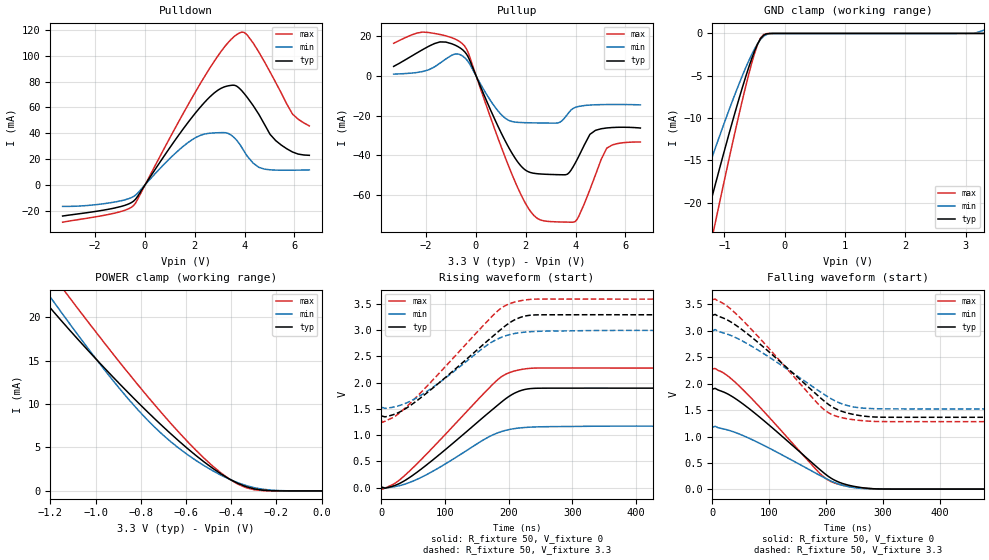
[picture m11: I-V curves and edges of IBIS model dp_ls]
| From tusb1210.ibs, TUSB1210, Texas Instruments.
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|   Model: dp_ls
|   Description:  DP in Low-Speed mode
[Model]   dp_ls
Model_type   I/O
Polarity   Non-Inverting
Enable   Active-Low
Vinh =   2.000
Vinl =   0.800
Vmeas =   1.650
Vref =   0
Cref =   300e-12
Rref =   10e6
|variable   typ   min   max
C_comp   8.000p   7.140p   8.830p
[Receiver Thresholds]
Vcross_low =   1.3
Vcross_high =   2.0
Vdiff_ac =   200m
Vdiff_dc =   50m
Tdiffslew_ac =   300n
[Temperature Range]   27   125   -40
[Voltage Range]   3.3   3.0   3.6
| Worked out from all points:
|   slope of the pulldown table from 0 to 0.495 V, typ, clamps not added: 33.9 ohm
|   slope of the pullup table from 0 to 0.495 V, typ, clamps not added: 33.6 ohm
|   GND clamp passes 1 mA (typ) near -0.43 V on its own axis
|   POWER clamp passes 1 mA (typ) near -0.38 V on its own axis
|   rising waveform, R_fixture 50, V_fixture 0: 20-80 % time 112ns typ, 95ns min, 107ns max; typ from 0.006 V to 1.9 V
|   rising waveform, R_fixture 50, V_fixture 3.3: 20-80 % time 112ns typ, 95ns min, 107ns max; typ from 1.36 V to 3.29 V
|   falling waveform, R_fixture 50, V_fixture 0: 20-80 % time 122ns typ, 123ns min, 115ns max; typ from 1.9 V to 0.006 V
|   falling waveform, R_fixture 50, V_fixture 3.3: 20-80 % time 122ns typ, 123ns min, 115ns max; typ from 3.29 V to 1.36 V
[GND Clamp]
| dp_ls
|Voltage   I(typ)   I(min)   I(max)
-3.3V     -79.58mA   -61.62mA   -98.43mA
-1.6V     -30.23mA   -22.96mA   -37.77mA
-1.55V    -28.83mA   -21.89mA   -36.03mA
-1.35V    -23.26mA   -17.65mA   -29.11mA
-1.3V     -21.89mA   -16.61mA   -27.4mA
-1.15V    -17.82mA   -13.52mA   -22.32mA
-850mV    -9.988mA   -7.653mA   -12.47mA
-600mV    -4.077mA   -3.29mA    -4.92mA
-450mV    -1.247mA   -1.203mA   -1.298mA
-350mV    -209.5uA   -330.6uA   -134.3uA
3.15V     -6.302nA   14.99uA    -5.951pA
3.3V      2.821nA    380.8uA    20.54pA
[POWER Clamp]
| dp_ls
|Voltage   I(typ)   I(min)   I(max)
-3.3V     105.3mA    103.2mA    112.5mA
-1.261V   22.96mA    24.54mA    27.34mA
-1.224V   21.79mA    23.18mA    26.03mA
-1.187V   20.66mA    21.84mA    24.74mA
-1.112V   18.45mA    19.18mA    22.17mA
-889.9mV  12.23mA    11.67mA    14.7mA
-741.6mV  8.388mA    7.416mA    10.01mA
-593.3mV  4.886mA    4.176mA    5.683mA
-444.9mV  1.953mA    1.81mA     2.063mA
-370.8mV  869.6uA    944uA      781.4uA
-296.6mV  225.9uA    362uA      131.2uA
0V        2.821nA    64.57nA    508.9pA
[Pulldown]
| dp_ls
|Voltage   I(typ)   I(min)   I(max)
-3.3V     -24.26mA   -16.79mA   -29.05mA
-450mV    -12.66mA   -9.071mA   -16.07mA
1.2V      34.26mA    24.05mA    43.44mA
2.1V      57.38mA    37.25mA    74.44mA
3.075V    75.05mA    40.48mA    103.9mA
3.45V     77.17mA    38.72mA    112.7mA
3.825V    74.32mA    30.96mA    118.1mA
4.125V    67.43mA    21.79mA    115.9mA
4.575V    54.67mA    13.52mA    103mA
5.25V     34.32mA    11.39mA    79.46mA
5.925V    25.45mA    11.32mA    54.89mA
6.6V      22.86mA    11.53mA    45.71mA
[Pullup]
| dp_ls
|Voltage   I(typ)   I(min)   I(max)
-3.3V     4.817mA    932uA      16.45mA
-2.37V    11.57mA    1.733mA    21.58mA
-1.44V    17.15mA    6.453mA    20.88mA
-450mV    12.17mA    9.19mA     15mA
1.125V    -31.43mA   -20.71mA   -39.28mA
1.875V    -46.18mA   -23.47mA   -61.42mA
2.55V     -49.29mA   -23.65mA   -72.25mA
3.6V      -49.71mA   -20.49mA   -73.55mA
3.975V    -44.09mA   -15.91mA   -73.34mA
4.575V    -29.39mA   -14.64mA   -57.2mA
5.25V     -26.17mA   -14.38mA   -36.36mA
6.6V      -26.2mA    -14.55mA   -33.25mA
[Ramp]
| dp_ls
|variable   typ   min   max
dV/dt_r   1.890/1.116e-07   1.168/9.496e-08   2.271/1.068e-07
dV/dt_f   1.930/1.221e-07   1.473/1.232e-07   2.310/1.155e-07
R_load =   50
[Rising Waveform]
| dp_ls
R_fixture =   50
V_fixture =   0
V_fixture_min =   0
V_fixture_max =   0
|Time   V(typ)   V(min)   V(max)
0s        5.744mV    4.231mV    7.585mV
1.656ns   4.577mV    8.553mV    -28.92mV
18.24ns   29.54mV    12.82mV    60.25mV
47.27ns   217.3mV    112.3mV    350.9mV
84.6ns    564.6mV    338.1mV    810.7mV
180ns     1.543V     1.03V      2.027V
196.6ns   1.705V     1.095V     2.168V
213.2ns   1.822V     1.132V     2.235V
250.5ns   1.895V     1.16V      2.28V
823.3ns   1.896V     1.172V     2.279V
[Rising Waveform]
| dp_ls
R_fixture =   50
V_fixture =   3.3
V_fixture_min =   3.0
V_fixture_max =   3.6
|Time   V(typ)   V(min)   V(max)
0s        1.364V     1.522V     1.282V
1.656ns   1.363V     1.528V     1.245V
18.24ns   1.389V     1.533V     1.336V
47.27ns   1.58V      1.659V     1.631V
84.6ns    1.935V     1.944V     2.099V
180ns     2.934V     2.817V     3.336V
196.6ns   3.099V     2.899V     3.48V
213.2ns   3.219V     2.945V     3.548V
250.5ns   3.294V     2.98V      3.593V
823.3ns   3.294V     2.996V     3.592V
[Falling Waveform]
| dp_ls
R_fixture =   50
V_fixture =   0
V_fixture_min =   0
V_fixture_max =   0
|Time   V(typ)   V(min)   V(max)
0s        1.896V     1.172V     2.279V
4.868ns   1.912V     1.196V     2.288V
19.46ns   1.844V     1.144V     2.205V
48.64ns   1.657V     1.042V     1.941V
194.5ns   323.1mV    232.1mV    245.7mV
209.1ns   207.3mV    154.7mV    144.2mV
228.6ns   112.2mV    77.31mV    77.78mV
262.6ns   32.87mV    18.1mV     26.36mV
296.6ns   7.605mV    6.292mV    8.666mV
963.5ns   5.744mV    4.231mV    7.585mV
[Falling Waveform]
| dp_ls
R_fixture =   50
V_fixture =   3.3
V_fixture_min =   3.0
V_fixture_max =   3.6
|Time   V(typ)   V(min)   V(max)
0s        3.294V     2.996V     3.592V
4.868ns   3.311V     3.025V     3.602V
19.46ns   3.241V     2.961V     3.517V
48.64ns   3.05V      2.832V     3.249V
194.5ns   1.688V     1.81V      1.524V
209.1ns   1.57V      1.712V     1.421V
228.6ns   1.473V     1.615V     1.354V
257.7ns   1.4V       1.545V     1.306V
296.6ns   1.366V     1.525V     1.283V
963.5ns   1.364V     1.522V     1.282V
